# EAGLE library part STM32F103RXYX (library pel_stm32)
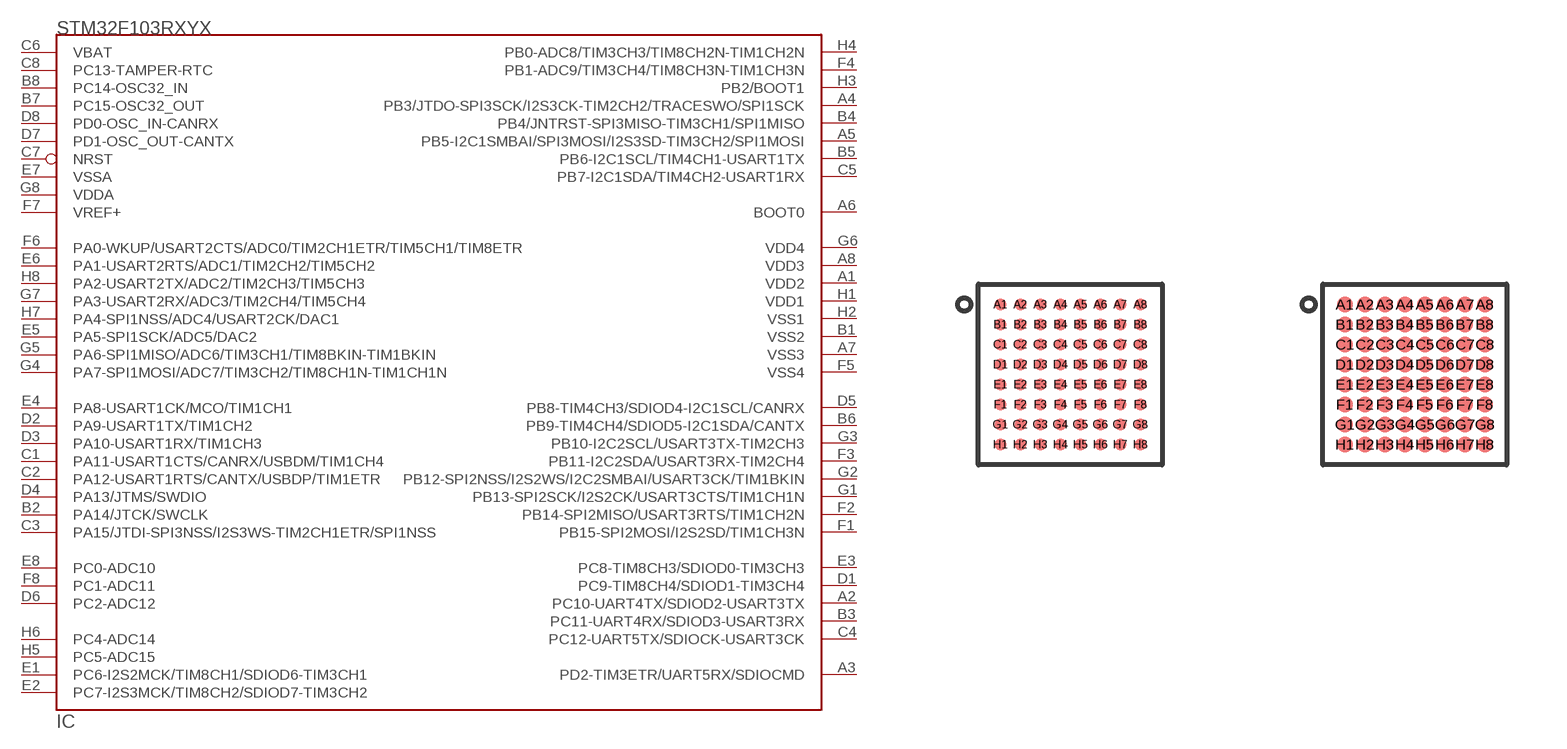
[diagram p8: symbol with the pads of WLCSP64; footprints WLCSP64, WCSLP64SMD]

Designator prefix IC

## STM32F103RXYX-NSMD  [WLCSP64]
A1  VDD2  sup
A2  PC10-UART4TX/SDIOD2-USART3TX
A3  PD2-TIM3ETR/UART5RX/SDIOCMD
A4  PB3/JTDO-SPI3SCK/I2S3CK-TIM2CH2/TRACESWO/SPI1SCK
A5  PB5-I2C1SMBAI/SPI3MOSI/I2S3SD-TIM3CH2/SPI1MOSI
A6  BOOT0  in
A7  VSS3  sup
A8  VDD3  sup
B1  VSS2  sup
B2  PA14/JTCK/SWCLK
B3  PC11-UART4RX/SDIOD3-USART3RX
B4  PB4/JNTRST-SPI3MISO-TIM3CH1/SPI1MISO
B5  PB6-I2C1SCL/TIM4CH1-USART1TX
B6  PB9-TIM4CH4/SDIOD5-I2C1SDA/CANTX
B7  PC15-OSC32_OUT
B8  PC14-OSC32_IN
C1  PA11-USART1CTS/CANRX/USBDM/TIM1CH4
C2  PA12-USART1RTS/CANTX/USBDP/TIM1ETR
C3  PA15/JTDI-SPI3NSS/I2S3WS-TIM2CH1ETR/SPI1NSS
C4  PC12-UART5TX/SDIOCK-USART3CK
C5  PB7-I2C1SDA/TIM4CH2-USART1RX
C6  VBAT  sup
C7  NRST
C8  PC13-TAMPER-RTC
D1  PC9-TIM8CH4/SDIOD1-TIM3CH4
D2  PA9-USART1TX/TIM1CH2
D3  PA10-USART1RX/TIM1CH3
D4  PA13/JTMS/SWDIO
D5  PB8-TIM4CH3/SDIOD4-I2C1SCL/CANRX
D6  PC2-ADC12
D7  PD1-OSC_OUT-CANTX  out
D8  PD0-OSC_IN-CANRX  in
E1  PC6-I2S2MCK/TIM8CH1/SDIOD6-TIM3CH1
E2  PC7-I2S3MCK/TIM8CH2/SDIOD7-TIM3CH2
E3  PC8-TIM8CH3/SDIOD0-TIM3CH3
E4  PA8-USART1CK/MCO/TIM1CH1
E5  PA5-SPI1SCK/ADC5/DAC2
E6  PA1-USART2RTS/ADC1/TIM2CH2/TIM5CH2
E7  VSSA  sup
E8  PC0-ADC10
F1  PB15-SPI2MOSI/I2S2SD/TIM1CH3N
F2  PB14-SPI2MISO/USART3RTS/TIM1CH2N
F3  PB11-I2C2SDA/USART3RX-TIM2CH4
F4  PB1-ADC9/TIM3CH4/TIM8CH3N-TIM1CH3N
F5  VSS4
F6  PA0-WKUP/USART2CTS/ADC0/TIM2CH1ETR/TIM5CH1/TIM8ETR
F7  VREF+
F8  PC1-ADC11
G1  PB13-SPI2SCK/I2S2CK/USART3CTS/TIM1CH1N
G2  PB12-SPI2NSS/I2S2WS/I2C2SMBAI/USART3CK/TIM1BKIN
G3  PB10-I2C2SCL/USART3TX-TIM2CH3
G4  PA7-SPI1MOSI/ADC7/TIM3CH2/TIM8CH1N-TIM1CH1N
G5  PA6-SPI1MISO/ADC6/TIM3CH1/TIM8BKIN-TIM1BKIN
G6  VDD4
G7  PA3-USART2RX/ADC3/TIM2CH4/TIM5CH4
G8  VDDA  sup
H1  VDD1  sup
H2  VSS1  sup
H3  PB2/BOOT1
H4  PB0-ADC8/TIM3CH3/TIM8CH2N-TIM1CH2N
H5  PC5-ADC15
H6  PC4-ADC14
H7  PA4-SPI1NSS/ADC4/USART2CK/DAC1
H8  PA2-USART2TX/ADC2/TIM2CH3/TIM5CH3

## STM32F103RXYX-SMD  [WCSLP64SMD]
Pads as for WLCSP64

## Footprint WLCSP64 (pad centres in mm)
smd 0.3 x 0.3: A1 -1.75,1.75; A2 -1.25,1.75; A3 -0.75,1.75; A4 -0.25,1.75; A5 0.25,1.75; A6 0.75,1.75; A7 1.25,1.75; A8 1.75,1.75; B1 -1.75,1.25; B2 -1.25,1.25; B3 -0.75,1.25; B4 -0.25,1.25; B5 0.25,1.25; B6 0.75,1.25; B7 1.25,1.25; B8 1.75,1.25; C1 -1.75,0.75; C2 -1.25,0.75; C3 -0.75,0.75; C4 -0.25,0.75; C5 0.25,0.75; C6 0.75,0.75; C7 1.25,0.75; C8 1.75,0.75; D1 -1.75,0.25; D2 -1.25,0.25; D3 -0.75,0.25; D4 -0.25,0.25; D5 0.25,0.25; D6 0.75,0.25; D7 1.25,0.25; D8 1.75,0.25; E1 -1.75,-0.25; E2 -1.25,-0.25; E3 -0.75,-0.25; E4 -0.25,-0.25; E5 0.25,-0.25; E6 0.75,-0.25; E7 1.25,-0.25; E8 1.75,-0.25; F1 -1.75,-0.75; F2 -1.25,-0.75; F3 -0.75,-0.75; F4 -0.25,-0.75; F5 0.25,-0.75; F6 0.75,-0.75; F7 1.25,-0.75; F8 1.75,-0.75; G1 -1.75,-1.25; G2 -1.25,-1.25; G3 -0.75,-1.25; G4 -0.25,-1.25; G5 0.25,-1.25; G6 0.75,-1.25; G7 1.25,-1.25; G8 1.75,-1.25; H1 -1.75,-1.75; H2 -1.25,-1.75; H3 -0.75,-1.75; H4 -0.25,-1.75; H5 0.25,-1.75; H6 0.75,-1.75; H7 1.25,-1.75; H8 1.75,-1.75

## Footprint WCSLP64SMD (pad centres in mm)
This design is based on: ST datasheet and Fairchild semi http://www.fairchildsemi.com/an/AN/AN-5026.pdf As well as our requirements from PCBCart to use 0.2mm via with 0.1mm annular ring...
smd 0.4 x 0.4: A1 -1.75,1.75; A2 -1.25,1.75; A3 -0.75,1.75; A4 -0.25,1.75; A5 0.25,1.75; A6 0.75,1.75; A7 1.25,1.75; A8 1.75,1.75; B1 -1.75,1.25; B2 -1.25,1.25; B3 -0.75,1.25; B4 -0.25,1.25; B5 0.25,1.25; B6 0.75,1.25; B7 1.25,1.25; B8 1.75,1.25; C1 -1.75,0.75; C2 -1.25,0.75; C3 -0.75,0.75; C4 -0.25,0.75; C5 0.25,0.75; C6 0.75,0.75; C7 1.25,0.75; C8 1.75,0.75; D1 -1.75,0.25; D2 -1.25,0.25; D3 -0.75,0.25; D4 -0.25,0.25; D5 0.25,0.25; D6 0.75,0.25; D7 1.25,0.25; D8 1.75,0.25; E1 -1.75,-0.25; E2 -1.25,-0.25; E3 -0.75,-0.25; E4 -0.25,-0.25; E5 0.25,-0.25; E6 0.75,-0.25; E7 1.25,-0.25; E8 1.75,-0.25; F1 -1.75,-0.75; F2 -1.25,-0.75; F3 -0.75,-0.75; F4 -0.25,-0.75; F5 0.25,-0.75; F6 0.75,-0.75; F7 1.25,-0.75; F8 1.75,-0.75; G1 -1.75,-1.25; G2 -1.25,-1.25; G3 -0.75,-1.25; G4 -0.25,-1.25; G5 0.25,-1.25; G6 0.75,-1.25; G7 1.25,-1.25; G8 1.75,-1.25; H1 -1.75,-1.75; H2 -1.25,-1.75; H3 -0.75,-1.75; H4 -0.25,-1.75; H5 0.25,-1.75; H6 0.75,-1.75; H7 1.25,-1.75; H8 1.75,-1.75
